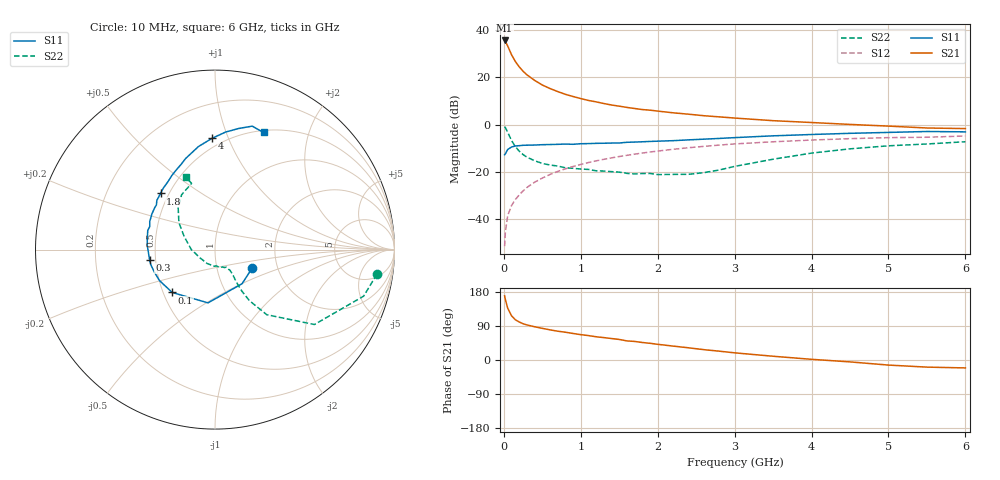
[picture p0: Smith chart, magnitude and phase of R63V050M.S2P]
! SIEMENS Small Signal Semiconductors
! BFR193
! Si NPN RF Bipolar Junction Transistor in SOT23
! VCE = 3 V  IC = 50 mA
! Common Emitter S-Parameters:  May  1996
# GHz  S  MA  R  50
!  f  S11  S21  S12  S22
! GHz  MAG  ANG  MAG  ANG  MAG  ANG  MAG  ANG
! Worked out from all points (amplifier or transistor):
!   36 points, 10 MHz to 6 GHz, reference 50 ohm
!   highest |S21| = 35.6 dB at 10 MHz (marker M1)
!   |S21| within 3 dB of that: start of sweep to 59.13 MHz
!   unconditionally stable (mu >= 1): 382.8 MHz to 1.861 GHz
!   at 250 MHz: K = 0.96, MSG = 25.3 dB, |S12| = -28.0 dB
!   at 1.4 GHz: K = 1.02, MAG = 10.2 dB, |S12| = -14.0 dB
!   at 6 GHz: K = 0.95, MSG = 1.6 dB, |S12| = -4.8 dB
!   S11 on the Smith chart (normalised r, x): 10 MHz: 1.48, -0.32; 100 MHz: 0.56, -0.30; 300 MHz: 0.46, -0.06; 1.8 GHz: 0.45, +0.35; 4 GHz: 0.43, +0.88; 6 GHz: 0.52, +1.36
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0.01  0.2313 -26.4  60.49 169.4  0.0027 82.7  0.913 -8.6
0.02  0.2427 -51.6  57.92 159.5  0.0054 78.9  0.8677 -17.4
0.05  0.2993 -97.5  46.29 136.8  0.0119 71.1  0.6936 -37.0
0.1  0.3374 -134.9  30.23 116.7  0.0195 69.8  0.4636 -51.5
0.15  0.3544 -150.9  21.66 106.1  0.0262 70.0  0.3435 -56.0
0.2  0.3607 -160.1  16.73 100.3  0.0328 72.5  0.2757 -57.1
0.25  0.3669 -166.4  13.51 95.7  0.0397 73.8  0.2336 -56.9
0.3  0.3689 -171.2  11.35 92.5  0.047 74.7  0.2063 -56.3
0.4  0.3716 -178.1  8.66 87.7  0.0609 74.8  0.1728 -54.7
0.5  0.378 176.6  6.912 83.5  0.0744 74.4  0.152 -54.3
0.6  0.3808 172.2  5.823 79.6  0.0886 73.6  0.1403 -54.1
0.8  0.3896 164.1  4.391 73.3  0.1169 71.6  0.1227 -56.4
1.1  0.3986 154.0  3.259 64.4  0.1583 68.0  0.1133 -62.3
1.4  0.4092 145.0  2.611 56.7  0.1988 63.7  0.1017 -71.8
1.8  0.4356 134.1  2.091 46.2  0.2515 57.6  0.0928 -92.1
2.2  0.4594 125.0  1.786 36.7  0.3019 51.5  0.089 -120.0
2.6  0.4948 115.6  1.549 27.3  0.3484 45.2  0.0968 -152.9
3.5  0.5816 99.1  1.217 9.9  0.4355 30.8  0.1864 157.0
4  0.6209 91.4  1.113 1.8  0.4739 23.7  0.2508 143.3
4.5  0.6572 84.9  1.014 -5.0  0.5073 16.6  0.3089 131.6
5.5  0.7185 73.2  0.852 -18.8  0.5431 2.8  0.3913 109.5
6  0.7063 67.5  0.828 -20.9  0.5772 -1.1  0.4363 111.9
